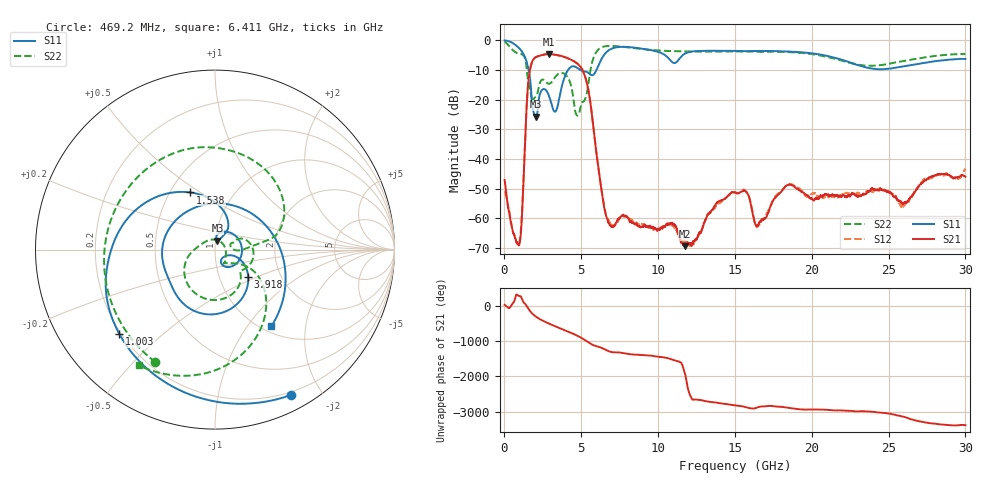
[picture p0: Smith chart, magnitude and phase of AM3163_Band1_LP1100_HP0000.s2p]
!Agilent Technologies,E8364B,MY43040894,A.07.50.67
!Agilent E8364B: A.07.50.67
!Date: Thursday, August 20, 2020 11:27:37
!Correction: S11(Full 2 Port(1,2))
!S21(Full 2 Port(1,2))
!S12(Full 2 Port(1,2))
!S22(Full 2 Port(1,2))
!S2P File: Measurements: S11, S21, S12, S22:
# Hz S  dB  R 50
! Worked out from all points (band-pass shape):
!   3201 points, 10 MHz to 30 GHz, reference 50 ohm
!   highest |S21| = -4.70 dB at 2.868 GHz (marker M1); lowest = -69.4 dB at 11.75 GHz (marker M2)
!   |S21| within 3 dB of the highest: 1.772 GHz to 4.693 GHz (2.921 GHz wide, 90.4 % of centre)
!   lowest |S11| = -25.8 dB at 2.034 GHz (marker M3), VSWR 1.11, Z = 51.1 + j5.09 ohm
!   |S11| at or under -10 dB: 1.571 GHz to 4.144 GHz (2.573 GHz wide, 90 % of centre); 4.912 GHz to 5.992 GHz (1.08 GHz wide, 19.8 % of centre)
!   |S22| runs from -25.4 to -0.5 dB; largest |S21 - S12| = 0.0082
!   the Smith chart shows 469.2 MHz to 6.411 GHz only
!   S11 on the Smith chart (normalised r, x): 469.2 MHz: 0.17, -1.64; 1.003 GHz: 0.19, -0.37; 1.538 GHz: 0.63, +0.46; 3.918 GHz: 1.37, -0.44; 6.411 GHz: 1.10, -1.31
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1e7  -0.10 -8.6  -47.09 21.3  -50.97 -113.9  -0.48 -18.9
4.692219e8  -0.78 -62.4  -62.83 21.2  -62.45 -57.7  -2.98 -117.9
1.003419e9  -2.97 -138.6  -67.79 -92.7  -67.03 -73.7  -4.60 131.2
1.537616e9  -9.20 113.3  -14.87 -74.2  -14.86 -74.3  -13.37 5.9
2.034325e9  -25.77 74.7  -5.75 53.2  -5.75 53.2  -19.07 21.3
2.512291e9  -16.51 4.5  -4.92 -69.0  -4.93 -69.0  -13.29 -15.3
2.868422e9  -18.38 -53.8  -4.70 -142.6  -4.71 -142.6  -14.68 -39.6
3.449478e9  -22.43 -25.8  -5.05 110.0  -5.07 109.9  -11.59 -67.2
3.918072e9  -12.41 -39.4  -5.67 27.0  -5.71 27.1  -11.38 -111.8
4.489756e9  -8.80 -101.4  -7.02 -78.5  -7.00 -78.3  -19.88 173.4
5.014581e9  -10.28 -147.2  -9.51 167.0  -9.49 166.9  -21.10 -52.1
5.783075e9  -11.67 77.5  -29.08 -36.3  -29.12 -36.3  -6.13 -57.6
6.410991e9  -5.52 -53.6  -53.84 -129.2  -53.53 -129.3  -2.25 -123.3
7.844888e9  -2.26 -175.7  -59.19 89.5  -59.24 87.7  -2.34 151.5
1.000979e10  -3.95 78.8  -63.40 -3.3  -63.96 3.1  -3.48 63.3
1.175296e10  -4.52 38.5  -69.38 -117.2  -67.93 142.0  -3.82 1.6
1.5005e10  -3.62 -71.8  -51.15 62.7  -51.46 63.4  -3.82 -92.5
1.647638e10  -3.65 -107.1  -62.45 7.6  -62.77 15.9  -3.91 -128.7
2.000958e10  -4.43 163.4  -53.28 -53.8  -51.82 -55.2  -4.69 136.3
2.274617e10  -7.98 60.6  -51.82 -99.5  -51.60 -99.8  -7.98 21.4
2.500479e10  -9.64 -62.3  -50.96 -168.1  -51.38 -169.0  -7.99 -92.4
3e10  -6.34 104.6  -46.04 -135.4  -43.31 -137.1  -4.63 102.0
